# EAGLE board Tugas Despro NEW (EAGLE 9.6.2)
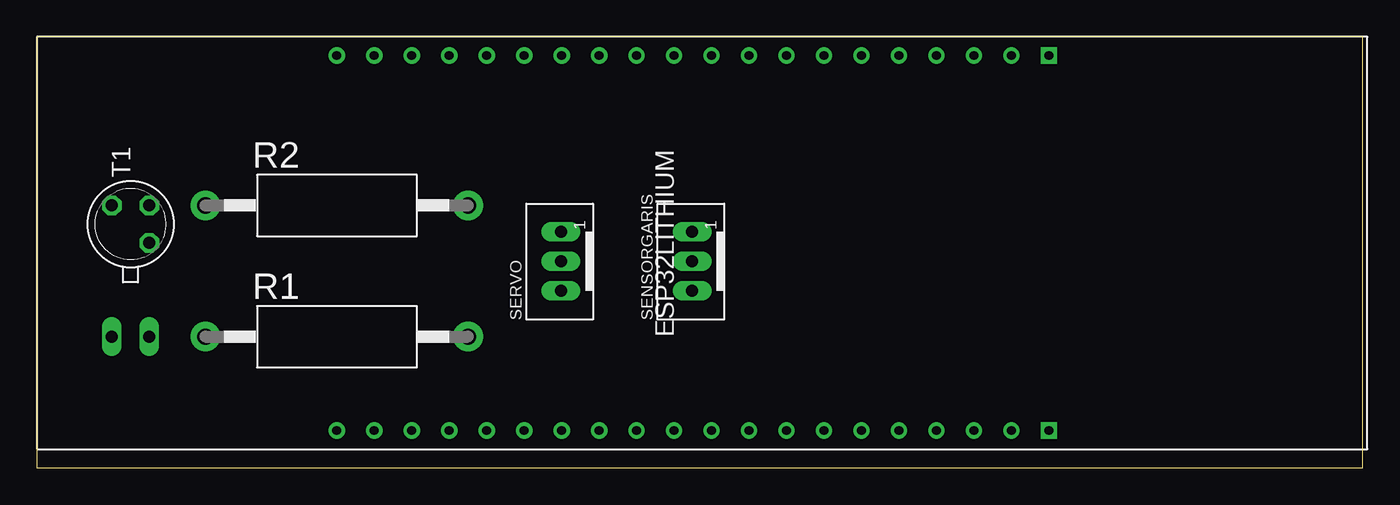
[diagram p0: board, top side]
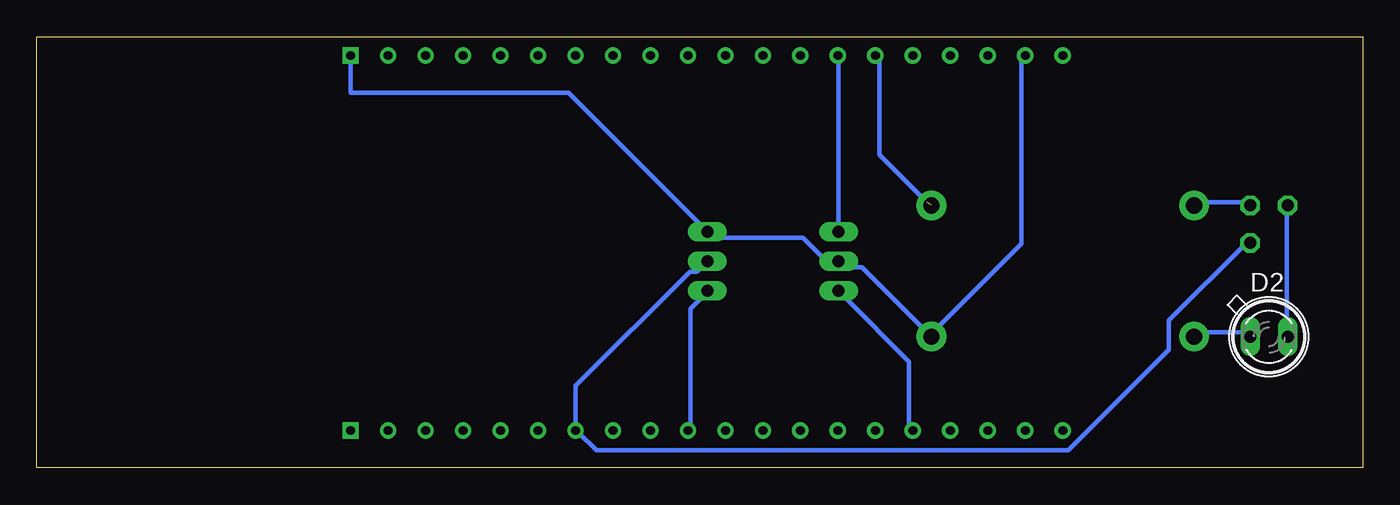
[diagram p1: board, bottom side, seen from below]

Size 89.84 x 29.2 mm. Coordinates in mm from the lower left corner, seen from the top.
Outline: 0,0 89.84,0 89.84,29.2 0,29.2 0,0
Copper layers (1*16): Top 0.035mm / dielectric 1.5mm / Bottom 0.035mm
Design rules "default *": minimum track width 0.3mm, minimum drill 0.6mm, track to track 0.5mm, track to pad 0.5mm, pad to pad 0.5mm, via to via 0.5mm, smd to smd 6mil, copper to edge 0.5mm, drill to drill 0.5mm, minimum pad ring 10mil, minimum via ring 8mil, stop-mask expansion 4mil, vias tented up to drill 0mil, thermal gap 10mil

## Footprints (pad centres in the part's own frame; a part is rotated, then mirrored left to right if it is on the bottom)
SFH482 = drill 0.813 long: A -1.27,0; K 1.27,0
AC01 = drill 1.1 pad 2: 1 -8.9,0; 2 8.9,0
JST_B3B-PH_HEADER = drill 0.8 long: P1 2.027,0.048; P2 0.028,0.048; P3 -1.972,0.048
TO18 = drill 0.813 octagon: 1 -1.27,-1.27; 2 1.27,-1.27; 3 1.27,1.27
ESP32LITHIUM = drill 0.6: 5V 25.4,-2.54; CLK 0,-2.54; CMD 25.4,-5.08; EN 25.4,-45.72; GND 0,-33.02; GND3 25.4,-15.24; GPIO0 0,-15.24; GPIO2 0,-12.7; GPIO4 0,-17.78; GPIO5 0,-25.4; GPIO12 25.4,-17.78; GPIO13 25.4,-12.7; GPIO14 25.4,-20.32; GPIO15 0,-10.16; GPIO16 0,-20.32; GPIO17 0,-22.86; GPIO18 0,-27.94; GPIO19 0,-30.48; GPIO21 0,-35.56; GPIO22 0,-43.18; GPIO23 0,-45.72; GPIO25 25.4,-27.94; GPIO26 25.4,-25.4; GPIO27 25.4,-22.86; GPIO32 25.4,-33.02; GPIO33 25.4,-30.48; GPIO34 25.4,-38.1; GPIO35 25.4,-35.56; NC 0,0; NC2 25.4,0; RX 0,-38.1; SD0 0,-5.08; SD1 0,-7.62; SD2 25.4,-10.16; SD3 25.4,-7.62; SVN 25.4,-40.64; SVP 25.4,-43.18; TX 0,-40.64 | drill 0.6 square: GND2 0,-48.26; VCC 25.4,-48.26

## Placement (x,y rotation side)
D2  SFH482  [SFH482]  6.35,8.89 0 bottom
R1  [AC01]  20.32,8.89 0 top
R2  [AC01]  20.32,17.78 0 top
SENSORGARIS  JST-PH_3-PIN_HEADER  [JST_B3B-PH_HEADER]  44.45,13.97 90 top
SERVO  JST-PH_3-PIN_HEADER  [JST_B3B-PH_HEADER]  35.56,13.97 90 top
T1  2N2222  [TO18]  6.35,16.51 90 top
U$5  ESP32LITHIUM  [ESP32LITHIUM]  20.32,2.54 90 top

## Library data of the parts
D2 = led
R1 R2 = resistor-power; OC_FARNELL: unknown; OC_NEWARK: unknown
SENSORGARIS SERVO = srg
T1 = transistor
U$5 = ESP32LITHIUM

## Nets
N$1: SENSORGARIS.P3 U$5.GPIO5
N$2: SENSORGARIS.P2 T1.1 U$5.GND
N$3: SERVO.P3 U$5.GPIO15
N$4: R2.2 U$5.GPIO13
N$5: R1.2 SERVO.P2
N$6: D2.A R1.1
N$7: SENSORGARIS.P1 U$5.VCC
N$8: D2.K T1.3
N$12: R2.1 T1.2
N$18: SERVO.P1 U$5.GND3

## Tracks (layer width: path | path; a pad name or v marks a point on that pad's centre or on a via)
N$1
  Bottom 0.3: U$5.GPIO5 45.53,2.8 45.53,10.8 44.73,11.6 SENSORGARIS.P3
N$2
  Bottom 0.3: T1.1 7.93,15.2 13.13,10 13.13,8 19.93,1.2 51.93,1.2 53.13,2.4 U$5.GND 53.34,5.56 45.6,13.3 45.1,13.3 SENSORGARIS.P2
N$3
  Bottom 0.3: U$5.GPIO15 30.73,2.8 30.73,7.2 35.13,11.6 SERVO.P3
N$4  (1 unrouted)
  Bottom 0.3: 29.53,18 32.73,21.2 32.73,27.6 U$5.GPIO13
N$5
  Bottom 0.3: 23.13,27.6 23.13,15.2 29.13,9.2 R1.2 33.93,13.6 35.13,13.6 SERVO.P2 35.53,14 36.33,14 37.93,15.6 44.33,15.6
N$6
  Bottom 0.3: D2.A 7.93,9.2 11.13,9.2 R1.1
N$7
  Bottom 0.3: SENSORGARIS.P1 53.8,25.4 68.58,25.4 U$5.VCC
N$8
  Bottom 0.3: D2.K 5.13,9.2 5.13,17.6 T1.3
N$12
  Bottom 0.3: T1.2 7.93,18 11.13,18 R2.1
N$18
  Bottom 0.3: U$5.GND3 35.53,27.6 35.53,16 SERVO.P1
